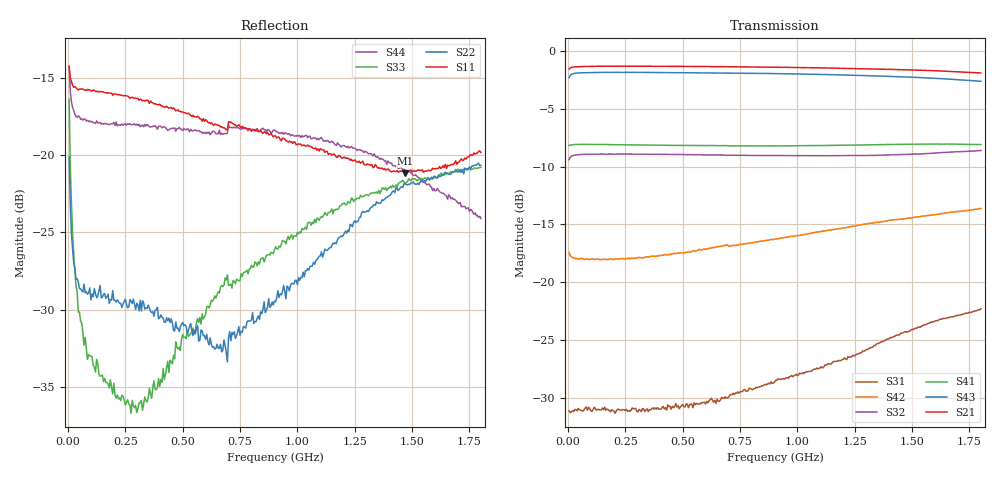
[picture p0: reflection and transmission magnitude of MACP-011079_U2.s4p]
!Agilent Technologies,E5071C,MY46110647,A.11.31
!Date: Tue Nov 07 14:16:53 2023
!Data & Calibration Information:
!MACP-011079 soldered onto PT-0003645 with F connectors, Calibration PT-0003653-TRL. Port1 (pin1) Port2 (pin6) Port3 (pin4) Port4 (pin3)
!Freq	S11:SOLT4(ON)	S12:SOLT4(ON)	S13:SOLT4(ON)	S14:SOLT4(ON)
!	S21:SOLT4(ON)	S22:SOLT4(ON)	S23:SOLT4(ON)	S24:SOLT4(ON)
!	S31:SOLT4(ON)	S32:SOLT4(ON)	S33:SOLT4(ON)	S34:SOLT4(ON)
!	S41:SOLT4(ON)	S42:SOLT4(ON)	S43:SOLT4(ON)	S44:SOLT4(ON)
!PortZ  Port1:75+j0  Port2:75+j0  Port3:75+j0  Port4:75+j0
!Above PortZ is port z conversion or system Z0 setting when saving the data.
!When reading, reference impedance value at option line is always used.
# Hz S MA R 75
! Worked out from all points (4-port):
!   360 points, 5 MHz to 1.8 GHz, reference 75 ohm
!   strongest paths, dB at 5 MHz, 455 MHz, 905 MHz, 1.355 GHz, 1.8 GHz:
!     S21: -1.6, -1.3, -1.4, -1.6, -1.9
!     S43: -2.3, -1.9, -2.0, -2.2, -2.6
!     S41: -8.2, -8.2, -8.2, -8.1, -8.1
!     S32: -9.4, -9.0, -9.0, -9.0, -8.6
!     S42: -17.4, -17.5, -16.3, -14.8, -13.6
!     S31: -31.1, -30.7, -28.5, -25.3, -22.3
!   lowest |S11| = -21.2 dB at 1.47 GHz (marker M1), VSWR 1.19, Z = 66.7 + j9.23 ohm
!   |S11| at or under -10 dB: start of sweep to end of sweep
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5000000  0.1938 161.6  0.8359 4.2  0.02753 25.5  0.3881 -177.5
         0.8351 4.1  0.09861 129.0  0.339 9.2  0.1364 174.0
         0.02778 25.3  0.3389 9.3  0.1516 118.0  0.7689 7.7
         0.3903 -177.4  0.1345 172.8  0.767 7.6  0.1936 149.8
2.5e7  0.1658 172.6  0.8523 0.6  0.02804 7.2  0.3935 179.1
       0.8525 0.7  0.04468 150.2  0.354 2.4  0.1288 176.6
       0.02764 6.5  0.3536 2.4  0.048 121.0  0.7981 1.5
       0.3935 179.0  0.1273 176.0  0.7984 1.5  0.1395 164.5
7e7  0.1625 174.5  0.857 -1.3  0.028 3.1  0.3944 175.4
     0.8567 -1.3  0.03827 169.4  0.3571 0.0  0.1273 175.9
     0.02808 2.6  0.3572 0.0  0.02425 128.8  0.805 -1.4
     0.3946 175.5  0.1256 175.2  0.8052 -1.4  0.1307 166.3
2.75e8  0.1534 167.9  0.8583 -7.2  0.02836 6.0  0.3919 161.1
        0.8588 -7.2  0.03373 -169.0  0.3577 -4.2  0.1297 166.4
        0.02802 3.3  0.3579 -4.2  0.01462 104.2  0.8073 -9.6
        0.3923 161.1  0.127 165.2  0.8079 -9.6  0.1253 145.9
6.95e8  0.1211 153.9  0.8543 -18.6  0.03133 12.1  0.3881 133.3
        0.8547 -18.7  0.02143 -126.3  0.3546 -11.0  0.1456 144.1
        0.03168 9.6  0.3541 -11.1  0.04102 32.4  0.8015 -25.2
        0.3894 133.3  0.1452 144.1  0.802 -25.2  0.1176 101.2
1.47e9  0.0874 128.2  0.8257 -40.4  0.05074 10.9  0.3905 83.8
        0.8287 -40.6  0.08052 -120.5  0.3567 -20.7  0.1829 99.1
        0.06122 10.1  0.357 -20.5  0.08091 -0.5  0.7719 -55.6
        0.395 84.2  0.1883 96.2  0.7717 -55.6  0.08943 44.1
1.8e9  0.1019 111.6  0.8009 -50.3  0.06871 2.4  0.3904 62.6
       0.8024 -50.6  0.09264 -128.3  0.3691 -25.2  0.2046 79.7
       0.07683 1.1  0.3711 -25.0  0.09129 -16.9  0.7399 -70.1
       0.3939 62.7  0.2085 76.5  0.7392 -70.0  0.06243 32.9
